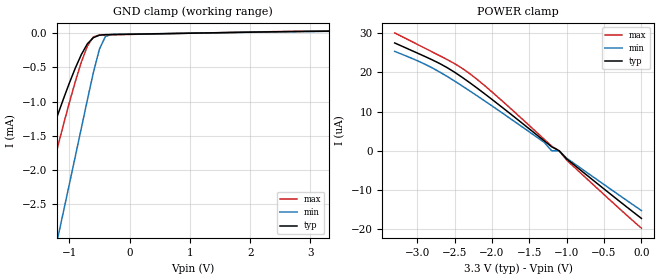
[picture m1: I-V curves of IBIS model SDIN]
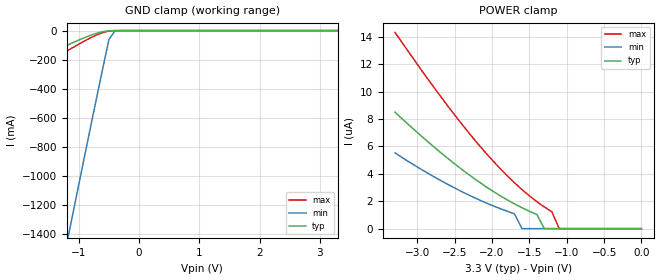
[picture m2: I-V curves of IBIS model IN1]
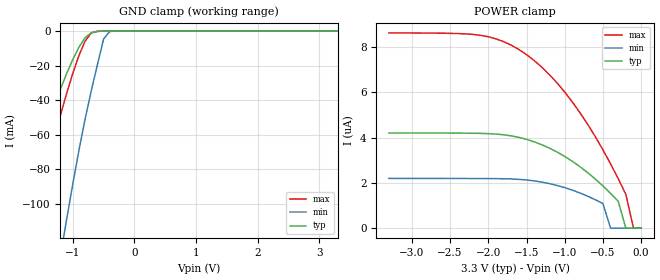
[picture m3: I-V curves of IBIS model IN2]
|IBIS model for MAX9242/44/46
|created by Maxim Integrated Products
|Package model is derived for 48 pin TSSOP package
[IBIS ver]   2.1
[File name]   max9242.ibs
[File Rev]   3.0
[Date]   Nov. 12, 2008
[Source]   From Maxim Spice models.
[Notes]   IBIS 2.1 does not support differetial buffers directly;
   the I-V and V-T curves are extracted by the
   methods recommended by members of IBIS committee.
[Disclaimer]   This file is for modeling purposes only.
[Copyright]   Copyright 2008 Maxim Integrated Products.
|   Component MAX9242
[Component]   MAX9242
[Manufacturer]   Maxim Integrated Products
[Package]
|variable   typ   min   max
R_pkg   0.085ohm   0.011ohm   0.098ohm
L_pkg   3.020nH   0.330nH   4.297nH
C_pkg   0.197pF   0.152pF   0.267pF
[Pin]   signal_name   model_name   r_pin   l_pin   c_pin
1   RxOUT17   DOUT   0.098   4.297nH   0.267pF
2   RxOUT18   DOUT   0.096   3.796nH   0.197pF
3   GND   GND   0.091   3.382nH   0.186pF
4   RxOUT19   DOUT   0.087   3.020nH   0.181pF
5   RxOUT20   DOUT   0.089   2.807nH   0.169pF
6   SSG   IN1   0.076   2.456nH   0.162pF
7   DCB   IN1   0.073   2.279nH   0.160pF
8   RxIN0-   SDIN   0.073   2.179nH   0.159pF
9   RxIN0+   SDIN   0.072   2.095nH   0.156pF
10   RxIN1-   SDIN   0.071   2.016nH   0.155pF
11   RXIN1+   SDIN   0.071   1.971nH   0.154pF
12   LVDSVCC   POWER   0.069		1.883nH		0.152pF
13   LVDSGND   GND   0.069		1.879nH		0.152pF
14   RxIN2-   SDIN   0.070   1.954nH   0.153pF
15   RxIN2+   SDIN   0.071   2.005nH   0.155pF
16   RxCLKIN-	SDIN   0.071   2.077nH   0.157pF
17   RxCLKIN+   SDIN   0.072   2.165nH   0.158pF
18   LVDSGND   GND   0.071   2.212nH   0.160pF
19   PLLGND   GND   0.073   2.342nH   0.162pF
20   PLLVCC   POWER   0.012   0.350nH   0.170pF
21   PLLGND   GND   0.086   2.984nH   0.181pF
22   PWRDWN*   IN2   0.090   3.307nH   0.186pF
23   RxCLKOUT	CLKOUT   0.095   3.745nH   0.197pF
24   RxOUT0   DOUT   0.097		4.284nH		0.266pF
25   GND   GND		0.097		4.261nH		0.266pF
26   RxOUT1   DOUT   0.094   3.704nH   0.197pF
27   RxOUT2   DOUT   0.090   3.295nH   0.186pF
28   VCCO   POWER   0.085   2.928nH   0.181pF
29   RxOUT3   DOUT   0.084   2.650nH   0.169pF
30   RxOUT4   DOUT   0.076   2.428nH   0.161pF
31   RxOUT5   DOUT   0.073   2.236nH   0.159pF
32   GND   GND   0.011   0.340nH   0.158pF
33   RxOUT6   DOUT   0.070   2.045nH   0.157pF
34   RxOUT7   DOUT   0.070   1.989nH   0.155pF
35   RxOUT8   DOUT   0.070   1.931nH   0.154pF
36   VCCO   POWER   0.070		1.898nH		0.152pF
37   RxOUT9   DOUT		0.070		1.912nH		0.152pF
38   GND   GND   0.071   1.978nH   0.154pF
39   RxOUT10   DOUT   0.070   1.976nH   0.156pF
40   RxOUT11   DOUT   0.071   2.076nH   0.157pF
41   RxOUT12   DOUT   0.071   2.144nH   0.157pF
42   VCC   POWER   0.011   0.330nH   0.160pF
43   DOUT13   DOUT   0.073   2.256nH   0.161pF
44   GND   GND   0.082   2.616nH   0.171pF
45   RxOUT14   DOUT   0.085   2.954nH   0.181pF
46   RxOUT15   DOUT   0.089   3.305nH   0.186pF
47   RxOUT16   DOUT   0.093   3.717nH   0.197pF
48   VCCO   POWER   0.097   4.252nH   0.267pF
[Diff_pin] inv_pin  vdiff  tdelay_typ
9   8   50mV   NA |Receiver Vth=+/-50mv
11   10   50mV   NA
| Models and submodels in the file (5): SDIN (Input), IN1 (Input), IN2 (Input), DOUT (Output), CLKOUT (Output)
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|   Model SDIN
[Model]   SDIN
Model_type   Input
|Signals   RxIN0-, RxIN0+, RxIN1-, RxIN1+
Vinh = 50mv
Vinl = -50mv
|   typ   min   max
C_comp   3.0pF   2.76pF   3.1pF
[Temperature Range]   25.00   85.00   -40
[Voltage Range]   3.30V   3.00V   3.60V
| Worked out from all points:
|   GND clamp passes 1 mA (typ) near -1.11 V on its own axis
[GND Clamp]
|Volts   I(typ)   I(min)   I(max)
-3.3V     -7.211mA   -11.48mA   -9.512mA
-1.8V     -2.838mA   -5.47mA    -3.875mA
-1.6V     -2.279mA   -4.659mA   -3.132mA
-1.5V     -2.006mA   -4.253mA   -2.765mA
-1.2V     -1.215mA   -3.03mA    -1.69mA
-1.1V     -969.7uA   -2.621mA   -1.348mA
-800mV    -314.2uA   -1.39mA    -424.5uA
-600mV    -66.62uA   -576.1uA   -55.97uA
-500mV    -30.67uA   -234.8uA   -28.22uA
-400mV    -23.01uA   -49.15uA   -25.72uA
-300mV    -21.5uA    -20.44uA   -24.38uA
3.3V      27.51uA    25.36uA    30.08uA
[POWER Clamp]
|Volts   I(typ)   I(min)   I(max)
-3.3V     27.51uA    25.36uA    30.08uA
-3V       24.96uA    23.01uA    27.18uA
-2.7V     22.28uA    20.11uA    24.27uA
-2.4V     18.78uA    16.58uA    21.08uA
-2.2V     16.03uA    14.06uA    18.25uA
-1.8V     10.15uA    8.835uA    11.66uA
-1.3V     2.539uA    2.158uA    2.939uA
-1.2V     1.017uA    0A         1.174uA
-1.1V     0A         0A         0A
-1V       -2.07uA    -1.886uA   -2.363uA
0V        -17.24uA   -15.24uA   -19.73uA
|   Model IN1
[Model]   IN1
Model_type   Input
|SIGNALS   SSG, DCB
Vinh = 2.0
Vinl = 0.8
|   typ   min   max
C_comp   1.5pF   1.35pF   1.65pF
[Temperature Range]   25.00   85.00   -40
[Voltage Range]   3.30V   3.00V   3.60V
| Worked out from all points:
|   GND clamp passes 1 mA (typ) near -0.47 V on its own axis
[GND Clamp]
|Volts   I(typ)   I(min)   I(max)
-3.3V     -532.9mA   -5.82A     -627.4mA
-2.3V     -335mA     -3.746A    -410.9mA
-1.2V     -102.8mA   -1.467A    -141.6mA
-1.1V     -83.42mA   -1.262A    -117.1mA
-700mV    -17.91mA   -452.8mA   -29.43mA
-500mV    -1.338mA   -60.21mA   -3.006mA
-400mV    -86.53uA   -2.531mA   -190.6uA
3.3V      8.499uA    5.535uA    14.32uA
[POWER Clamp]
|Volts   I(typ)   I(min)   I(max)
-3.3V     8.499uA    5.535uA    14.32uA
-2.8V     6.064uA    3.858uA    10.47uA
-2.4V     4.303uA    2.689uA    7.594uA
-2.2V     3.505uA    2.168uA    6.26uA
-2V       2.771uA    1.696uA    5.015uA
-1.7V     1.808uA    1.085uA    3.348uA
-1.6V     1.527uA    0A         2.854uA
-1.4V     1.03uA     0A         1.969uA
-1.3V     0A         0A         1.581uA
-1.2V     0A         0A         1.233uA
-1.1V     0A         0A         0A
0V        0A         0A         0A
|   Model IN2
[Model]   IN2
Model_type   Input
|Signals   PWRDWN*
Vinh = 2.0
Vinl = 0.8
|   typ   min   max
C_comp   2.36pF   2.12pF   2.6pF
[Temperature Range]   25.00   85.00   -40
[Voltage Range]   3.30V   3.00V   3.60V
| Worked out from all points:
|   GND clamp passes 1 mA (typ) near -0.70 V on its own axis
[GND Clamp]
|Volts   I(typ)   I(min)   I(max)
-3.3V     -261.4mA   -614.8mA   -335.9mA
-2V       -118.7mA   -311.2mA   -160.3mA
-1.9V     -107.5mA   -287.9mA   -146.1mA
-1.7V     -85.29mA   -241.7mA   -117.7mA
-1.2V     -33.6mA    -130.2mA   -48.68mA
-1.1V     -24.63mA   -109.1mA   -36.15mA
-900mV    -9.3mA     -69mA      -14.1mA
-800mV    -3.827mA   -50.87mA   -5.796mA
-700mV    -960.7uA   -34.54mA   -1.068mA
-500mV    -35.48uA   -4.576mA   -6.34uA
-400mV    -2.735uA   -183.1uA   -3.44uA
3.3V      4.203uA    2.196uA    8.618uA
[POWER Clamp]
|Volts   I(typ)   I(min)   I(max)
-3.3V     4.203uA    2.196uA    8.618uA
-2V       4.171uA    2.188uA    8.448uA
-1.7V     4.073uA    2.171uA    8.076uA
-1.4V     3.811uA    2.087uA    7.4uA
-1V       3.166uA    1.788uA    6.006uA
-700mV    2.451uA    1.411uA    4.585uA
-500mV    1.864uA    1.085uA    3.457uA
-400mV    1.536uA    0A         2.839uA
-300mV    1.186uA    0A         2.184uA
-200mV    0A         0A         1.493uA
-100mV    0A         0A         0A
0V        0A         0A         0A
